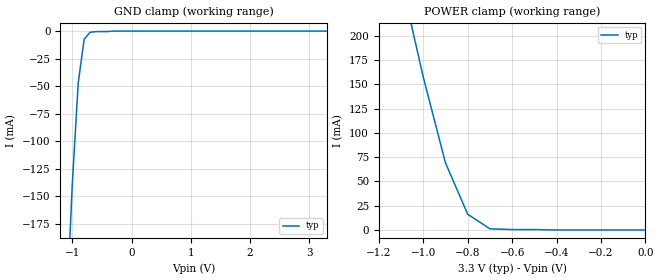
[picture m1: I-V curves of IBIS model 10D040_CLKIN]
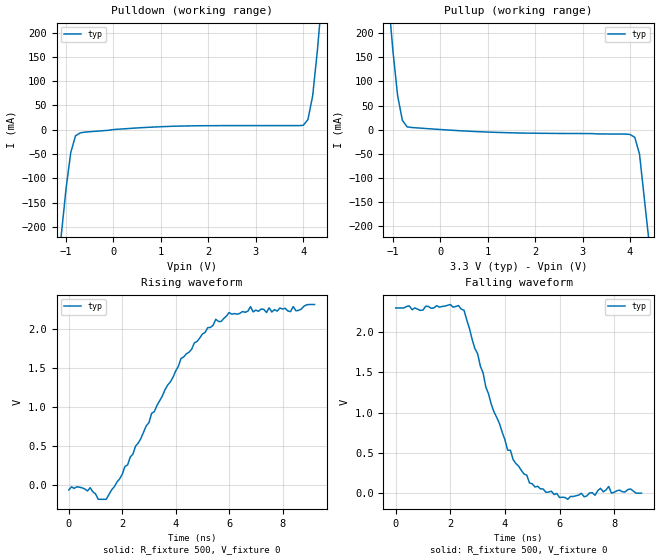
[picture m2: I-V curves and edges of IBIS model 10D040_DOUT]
|   National Semiconductor Corporation
|   Data Conversion Products Group
|   IBIS Model of ADC10D040
|   48 Pin TQFP Package
[IBIS Ver]   3.2
[File name]   adc10d040.ibs
[File Rev]   1.1
[Date]   08/17/2006
[Source]   bench to Ibis Conversion
[Notes]   File created by RC from ADC10D040 model
[Disclaimer]
(C) Copyright National Semiconductor Corporation 2006
   All rights reserved
   National Semiconductor Corporation hereby grants
the user of this IBIS model a non-exclusive, nontransferable
license to use this IBIS model under the following terms.
Before using this IBIS model, the user should read this
license.  If the user does not accept these terms,  the
IBIS model should be returned to National within 30 days.
   The user is granted this license only to use the
IBIS model and is not granted rights to sell, load, rent,
lease or license the IBIS model in whole or in part, or in
modified form to anyone other than user. User may modify
the IBIS model to suit its specific applications but rights
to derivative works and such modifications shall belong to
National.
   This IBIS model is provided on an "AS IS" basis and
National makes absolutely no warranty with respect to the
information contained herein.NATIONAL DISCLAIMS AND CUSTOMER
WAIVES ALL WARRANTIES, EXPRESS OR IMPLIED, INCLUDING
WARRANTIES OF MERCHANTABILITY OR FITNESS FOR A PARTICULAR
PURPOSE. The entire risk as to quality and performance is
with the Customer. ACCORDINGLY, IN NO EVENT SHALL THE
COMPANY BE LIABLE FOR ANY DAMAGES, WHETHER IN CONTRACT OR
TORT,INCLUDING ANY LOST PROFITS OR OTHER INCIDENTAL,
CONSEQUENTIAL, EXEMPLARY, OR PUNITIVE DAMAGES ARISING OUT
OF THE USE OR APPLICATION OF THE IBIS model provided in
this package.Further, National reserves the right to make
changes without notice to any product herein to improve
reliability, function, or design. National does not convey
any license under patent rights or any other intellectual
property rights, including those of third parties.
   National is not obligated to provide maintenance or support
for the licensed IBIS model.
Contact National at ATTN:DCS APPLICATIONS/IBIS MODELS.
2900 Semiconductor Drive, M/S D3-739, Santa Clara, CA 95052-8090
[Copyright]   Copyright 2006, National Semiconductor, All Rights Reserved
[Component]   ADC10D040
[Manufacturer]  National Semiconductor Corp
[Package]
|   typ   min   max
R_pkg   390m   350m   450m
L_pkg   3.476nH   3.137n   3.995n
C_pkg   0.15pF   0.124pF   0.228pF
[Pin]   signal_name   model_name   R_pin   L_pin   C_pin
1   VREF   NC
2   OS   NC
3   AGND   GND
4   VD   POWER
5   DGND   GND
6   VDR   POWER
7   DRGND   GND
8   I9   10D040_DOUT
9   I8   10D040_DOUT
10   I7   10D040_DOUT
11   I6   10D040_DOUT
12   I5   10D040_DOUT
13   I4   10D040_DOUT
14   I3   10D040_DOUT
15   I2   10D040_DOUT
16   I1   10D040_DOUT
17   I0   10D040_DOUT
18   Q9   10D040_DOUT
19   Q8   10D040_DOUT
20   Q7   10D040_DOUT
21   Q6   10D040_DOUT
22   Q5   10D040_DOUT
23   Q4   10D040_DOUT
24   Q3   10D040_DOUT
25   Q2   10D040_DOUT
26   Q1   10D040_DOUT
27   Q0   10D040_DOUT
28   IQ   NC
29   DRGND   GND
30   VDR   POWER
31   OC   NC
32   OF   NC
33   CLK   10D040_CLKIN
34   STBY   NC
35   PD   NC
36   GAIN   NC
37   Q+   NC
38   Q-   NC
39   AGND   GND
40   VA   POWER
41   VA   POWER
42   AGND   GND
43   VRP   NC
44   VRN   NC
45   VCMO   NC
46   AGND   GND
47   I-   NC
48   I+   NC
| Models and submodels in the file (2): 10D040_CLKIN (Input), 10D040_DOUT (Output)
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|   Clock Input MODEL
[Model]   10D040_CLKIN
Model_type Input
Vinh=2.0
Vinl=1.0
|   TYP   MIN   MAX
C_comp   0.1p   0.1p   0.1p
[Temperature Range] 27   NA   NA
[Voltage Range]   3.3   NA   NA
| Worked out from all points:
|   GND clamp passes 1 mA (typ) near -0.68 V on its own axis
|   POWER clamp passes 1 mA (typ) near -0.67 V on its own axis
[GND Clamp]
|V(groundclamp)   I(typ)   I(min)   I(max)
-3.3V     -2.883A    NA         NA
-1.1V     -257.6mA   NA         NA
-1V       -138.8mA   NA         NA
-900mV    -47mA      NA         NA
-800mV    -7.4mA     NA         NA
-700mV    -1.1mA     NA         NA
-300mV    0A         NA         NA
3.3V      0A         NA         NA
[POWER Clamp]
|V(table)   I(typ)   I(min)   I(max)
-3.3V     2.274A     NA         NA
-1.1V     258.2mA    NA         NA
-1V       157.5mA    NA         NA
-900mV    69.1mA     NA         NA
-800mV    16.2mA     NA         NA
-700mV    1.2mA      NA         NA
-400mV    0A         NA         NA
0V        0A         NA         NA
|   Driver Output MODEL
[Model]   10D040_DOUT
Model_type Output
Polarity Non-Inverting
|   TYP   MIN   MAX
C_comp   0.1p   0.1p   0.1p
[Temperature Range] 27   NA   NA
[Voltage Range]   3.3   NA   NA
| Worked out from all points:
|   slope of the pulldown table from 0 to 0.495 V, typ, clamps not added: 151 ohm
|   slope of the pullup table from 0 to 0.495 V, typ, clamps not added: 166 ohm
|   falling waveform, R_fixture 500, V_fixture 0: 20-80 % time 1.4ns typ, NA min, NA max; typ from 2.3 V to 0 V
|   rising waveform, R_fixture 500, V_fixture 0: 20-80 % time 2.37ns typ, NA min, NA max; typ from -0.06 V to 2.31 V
[Pullup]
|Vtable   I(typ)   I(min)   I(max)
-3.3V     2.704A     NA         NA
-1.1V     277.8mA    NA         NA
-1V       164.2mA    NA         NA
-900mV    70.3mA     NA         NA
-800mV    19.6mA     NA         NA
-700mV    6mA        NA         NA
4V        -9.8mA     NA         NA
4.1V      -15.8mA    NA         NA
4.2V      -50.5mA    NA         NA
4.3V      -141.2mA   NA         NA
4.4V      -231.9mA   NA         NA
6.6V      -2.227A    NA         NA
[Pulldown]
|V(pulldown)   I(typ)   I(min)   I(max)
-3.3V     -2.415A    NA         NA
-1.1V     -217mA     NA         NA
-1V       -122mA     NA         NA
-900mV    -46.9mA    NA         NA
-800mV    -12.6mA    NA         NA
-700mV    -6.4mA     NA         NA
4V        9mA        NA         NA
4.1V      20.8mA     NA         NA
4.2V      69.4mA     NA         NA
4.3V      163.1mA    NA         NA
4.4V      276.3mA    NA         NA
6.6V      2.736A     NA         NA
[Ramp]
|   TYP   MIN   MAX
dV/dt_r   1.9/3.2E-9   NA   NA
dV/dt_f   1.9/1.96E-9   NA   NA
R_load=500
[Falling Waveform]
R_fixture=500
V_fixture=0
|Time   V(typ)   V(min)   V(max)
0s        2.3V       NA         NA
2ns       2.343V     NA         NA
2.5ns     2.273V     NA         NA
3.3ns     1.318V     NA         NA
4.1ns     533mV      NA         NA
4.9ns     126mV      NA         NA
6.3ns     -77mV      NA         NA
7.8ns     83mV       NA         NA
7.9ns     1mV        NA         NA
9ns       0V         NA         NA
[Rising Waveform]
R_fixture=500
V_fixture=0
|Time   V(typ)   V(min)   V(max)
0s        -60mV      NA         NA
800ps     -31mV      NA         NA
1.1ns     -179mV     NA         NA
1.4ns     -180mV     NA         NA
2.2ns     260mV      NA         NA
4.2ns     1.62V      NA         NA
5.5ns     2.121V     NA         NA
6.8ns     2.283V     NA         NA
7.4ns     2.207V     NA         NA
9.2ns     2.31V      NA         NA
